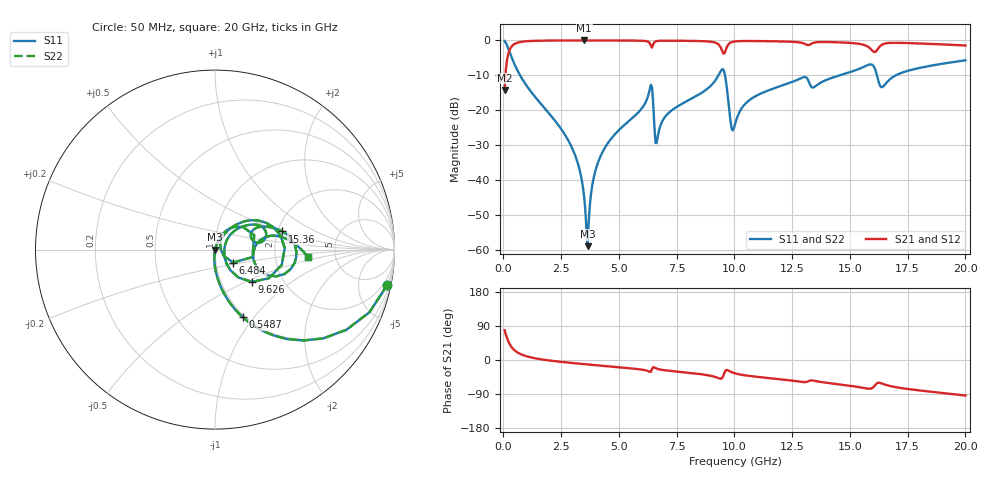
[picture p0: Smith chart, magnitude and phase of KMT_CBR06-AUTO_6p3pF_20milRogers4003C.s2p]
! Data measured by Modelithics Inc. support@modelithics.com 813-866-6335
! KEMET CBR06-AUTO 6.3pF, Pad Width= 0.851mm, Pad Length= 0.64mm, Pad Gap= 0.62mm, 20mil Rogers 4003C substrate Data, January 2022
# hz S ma R 50
! 2 Port Network Data from SP1.SP block
! freq  magS11  angS11  magS21  angS21  magS12  angS12  magS22  angS22
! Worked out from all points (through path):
!   401 points, 50 MHz to 20 GHz, reference 50 ohm
!   highest |S21| = -0.01 dB at 3.491 GHz (marker M1); lowest = -14.2 dB at 50 MHz (marker M2)
!   group delay of S21, straight-line fit = 14.5 ps
!   lowest |S11| = -58.8 dB at 3.641 GHz (marker M3), VSWR 1.00, Z = 50.1 + j0.00746 ohm
!   |S11| at or under -10 dB: 722.9 MHz to 9.306 GHz (8.584 GHz wide, 171 % of centre); 9.593 GHz to 14.55 GHz (4.958 GHz wide, 41.1 % of centre); 16.17 GHz to 16.98 GHz (814.2 MHz wide, 4.91 % of centre)
!   |S22| runs from -58.8 to -0.2 dB; largest |S21 - S12| = 0
!   S11 on the Smith chart (normalised r, x): 50 MHz: 0.97, -9.87; 548.8 MHz: 0.97, -0.88; 6.484 GHz: 1.21, -0.18; 9.626 GHz: 1.40, -0.54; 15.36 GHz: 2.11, +0.50; 20 GHz: 3.12, -0.35
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5e7  0.9806 -11.5  0.1959 78.5  0.1959 78.5  0.9806 -11.5
2.495e8  0.7065 -45.8  0.7072 44.1  0.7072 44.1  0.7065 -45.8
5.4875e8  0.4074 -67.7  0.9126 22.3  0.9126 22.3  0.4074 -67.7
2.74325e9  0.04063 -95.2  0.9981 -6.5  0.9981 -6.5  0.04063 -95.2
3.391625e9  0.01011 -94.3  0.9988 -10.4  0.9988 -10.4  0.01011 -94.3
3.491375e9  0.00594 -90.4  0.9988 -10.9  0.9988 -10.9  0.00594 -90.4
3.641e9  0.001151 3.7  0.9988 -11.8  0.9988 -11.8  0.001151 3.7
3.94025e9  0.01218 71.1  0.9986 -13.4  0.9986 -13.4  0.01218 71.1
4.389125e9  0.02917 71.7  0.9982 -15.8  0.9982 -15.8  0.02917 71.7
6.33425e9  0.2003 39.1  0.9144 -31.2  0.9144 -31.2  0.2003 39.1
6.483875e9  0.1245 -35.6  0.8799 -18.8  0.8799 -18.8  0.1245 -35.6
6.73325e9  0.05141 52.5  0.987 -24.5  0.987 -24.5  0.05141 52.5
9.227e9  0.2852 34.8  0.9128 -45.9  0.9128 -45.9  0.2852 34.8
9.626e9  0.2736 -41.1  0.7322 -26.9  0.7322 -26.9  0.2736 -41.1
9.875375e9  0.05601 -23.4  0.9442 -32.0  0.9442 -32.0  0.05601 -23.4
1.0025e10  0.0634 26.1  0.9677 -35.2  0.9677 -35.2  0.0634 26.1
1.107238e10  0.1699 42.7  0.9785 -45.0  0.9785 -45.0  0.1699 42.7
1.336662e10  0.2124 16.5  0.9079 -53.9  0.9079 -53.9  0.2124 16.5
1.536162e10  0.3878 15.2  0.897 -71.2  0.897 -71.2  0.3878 15.2
1.610975e10  0.3722 -23.6  0.6892 -64.9  0.6892 -64.9  0.3722 -23.6
1.670825e10  0.2739 13.1  0.9208 -68.2  0.9208 -68.2  0.2739 13.1
2e10  0.5198 -4.5  0.8461 -93.7  0.8461 -93.7  0.5198 -4.5
